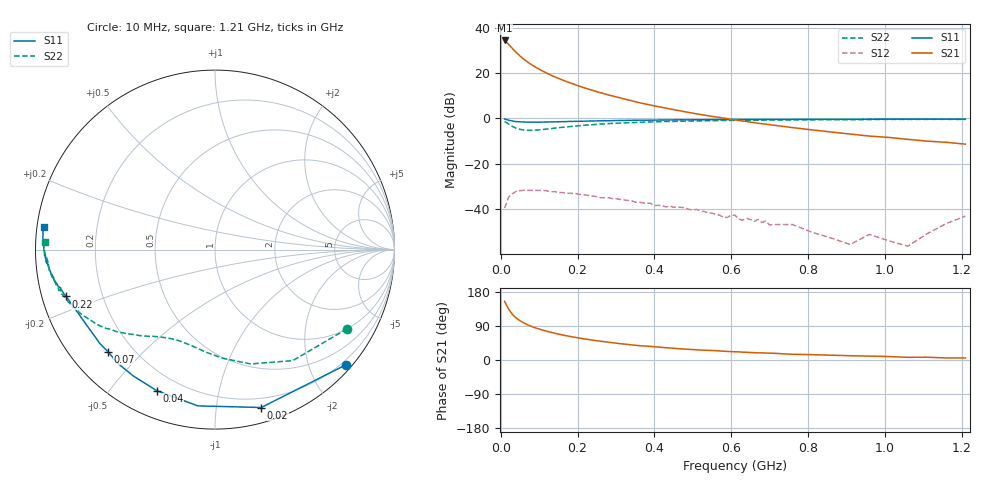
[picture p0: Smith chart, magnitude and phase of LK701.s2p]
! Date: Wed May 20 11:17:12 1998
!  POLYFET RF DEVICES
!  LP701/LK701
!  28Vdc		200ma
# MHZ  S  MA  R  50.0000
! SCATTERING PARAMETERS :
! Freq=MHz Mag[s11] Ang[s11] Mag[s21] Ang[s21] Mag[s12] Ang[s12] Mag[s22] Ang[s22]
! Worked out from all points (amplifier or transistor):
!   81 points, 10 MHz to 1.21 GHz, reference 50 ohm
!   highest |S21| = 34.4 dB at 10 MHz (marker M1)
!   |S21| within 3 dB of that: start of sweep to 27.33 MHz
!   unconditionally stable (mu >= 1): 589.082 MHz to 590.3746 MHz; 616.4 MHz to end of sweep
!   at 140 MHz: K = 0.09, MSG = 25.3 dB, |S12| = -32.3 dB
!   at 410 MHz: K = 0.38, MSG = 21.8 dB, |S12| = -38.3 dB
!   at 1.21 GHz: K = 2.43, MAG = 9.2 dB, |S12| = -43.1 dB
!   S11 on the Smith chart (normalised r, x): 10 MHz: 0.12, -2.64; 20 MHz: 0.12, -1.33; 40 MHz: 0.12, -0.66; 70 MHz: 0.11, -0.40; 220 MHz: 0.07, -0.15; 1.21 GHz: 0.02, +0.07
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10  0.9707 -41.5  52.35 154.6  0.01051 64.8  0.8589 -30.9
20  0.9168 -73.7  43.33 134.9  0.01811 43.2  0.7551 -55.0
30  0.8758 -96.3  35.02 120.9  0.02167 32.0  0.667 -72.7
40  0.8502 -112.5  28.58 111.1  0.02468 23.7  0.6077 -85.7
50  0.8385 -122.7  23.87 103.7  0.02541 14.9  0.5744 -94.8
60  0.8334 -130.5  20.27 97.9  0.02601 9.7  0.5541 -101.9
70  0.8244 -136.4  17.48 92.8  0.02602 6.2  0.5469 -107.4
80  0.828 -140.9  15.31 88.5  0.02589 0.3  0.5458 -111.7
100  0.8273 -147.3  12.16 81.7  0.02569 -5.0  0.5599 -118.4
130  0.8368 -153.4  9.042 73.2  0.02409 -12.3  0.5952 -125.8
170  0.8502 -158.6  6.548 64.1  0.02232 -20.9  0.648 -132.9
210  0.8665 -161.9  4.965 56.9  0.02083 -26.0  0.6965 -138.4
220  0.8686 -162.5  4.652 55.4  0.02052 -26.8  0.7082 -139.5
300  0.8983 -167.0  2.993 44.5  0.01702 -35.6  0.7819 -148.2
410  0.919 -171.3  1.821 34.2  0.01213 -36.7  0.8443 -157.0
610  0.9432 -176.6  0.9277 21.7  0.00735 -48.5  0.9042 -167.0
810  0.9542 179.3  0.5583 14.1  0.00309 -38.7  0.9311 -173.7
910  0.9571 177.7  0.4511 11.3  0.00166 81.1  0.9336 -175.9
960  0.9589 176.8  0.4074 10.3  0.00276 67.9  0.9408 -177.5
1010  0.9618 176.0  0.3808 9.2  0.002 77.4  0.9508 -178.5
1060  0.9612 175.0  0.3449 7.0  0.00152 86.8  0.9501 -179.6
1210  0.9627 172.5  0.2705 5.4  0.00699 105.9  0.9482 177.4
